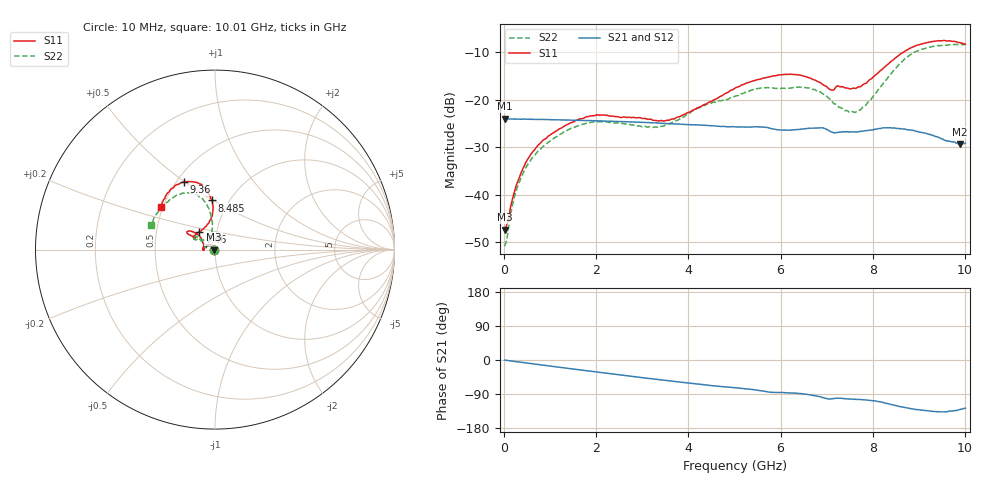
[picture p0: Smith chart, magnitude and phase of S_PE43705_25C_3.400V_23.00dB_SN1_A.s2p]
! Device ID: PE43705
! Serial: 1
! Insertion: A
! Impedance: 50 ohm
! Temp: 25C
! VDD: 3.400V
! Attenuation Step: 23.00dB
#  Hz  S  RI  R  50
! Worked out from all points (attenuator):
!   401 points, 10 MHz to 10.01 GHz, reference 50 ohm
!   highest |S21| = -24.02 dB at 10 MHz (marker M1); lowest = -29.3 dB at 9.885 GHz (marker M2)
!   lowest |S11| = -47.4 dB at 10 MHz (marker M3), VSWR 1.01, Z = 49.6 + j0.0438 ohm
!   |S11| at or under -10 dB: start of sweep to 8.665 GHz
!   |S22| runs from -50.8 to -8.3 dB; largest |S21 - S12| = 0.001
!   S11 on the Smith chart (normalised r, x): 10 MHz: 0.99, +0.00; 7.46 GHz: 0.82, +0.16; 8.485 GHz: 0.83, +0.49; 9.36 GHz: 0.55, +0.50; 10.01 GHz: 0.49, +0.27
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1e7  -0.00426 0.000441  0.0629 -0.000248  0.063 -0.000261  -0.00284 0.000469
2.6e8  -0.00556 0.0111  0.0624 -0.00478  0.0623 -0.00473  -0.00361 0.0104
5.35e8  -0.0124 0.0212  0.0616 -0.00955  0.0616 -0.00946  -0.00964 0.0192
1.01e9  -0.0331 0.0274  0.0592 -0.0173  0.0592 -0.0173  -0.0277 0.0245
1.685e9  -0.0608 0.0173  0.0541 -0.0271  0.0541 -0.0271  -0.0522 0.0168
2.085e9  -0.0685 0.00614  0.0503 -0.0323  0.0503 -0.0322  -0.0581 0.00856
3.36e9  -0.0597 0.00424  0.035 -0.0445  0.0351 -0.0446  -0.05 0.0129
3.86e9  -0.063 0.0271  0.0285 -0.0472  0.0286 -0.0471  -0.0586 0.0278
4.385e9  -0.0727 0.053  0.022 -0.049  0.0221 -0.049  -0.0746 0.0479
5.01e9  -0.0995 0.0874  0.0147 -0.0497  0.0151 -0.0496  -0.0886 0.0634
5.535e9  -0.129 0.1006  0.00857 -0.0511  0.00868 -0.051  -0.1083 0.0743
5.985e9  -0.1513 0.1026  0.0036 -0.0479  0.00359 -0.0478  -0.11 0.0713
6.685e9  -0.1432 0.082  -0.00276 -0.0501  -0.00292 -0.05  -0.1144 0.0587
7.085e9  -0.1096 0.0646  -0.0102 -0.045  -0.0101 -0.0452  -0.0841 0.0555
7.46e9  -0.0883 0.0984  -0.0101 -0.045  -0.0101 -0.0447  -0.0498 0.0575
7.785e9  -0.0449 0.1365  -0.012 -0.0452  -0.0115 -0.0452  -0.0276 0.079
8.36e9  -0.0109 0.244  -0.0223 -0.0455  -0.0223 -0.0456  -0.0198 0.1788
8.485e9  -0.0172 0.2737  -0.0249 -0.0435  -0.025 -0.0436  -0.0289 0.2102
8.885e9  -0.0692 0.3537  -0.03 -0.0367  -0.0295 -0.0365  -0.0908 0.297
9.36e9  -0.1718 0.3752  -0.0296 -0.0283  -0.0297 -0.0284  -0.1986 0.3067
9.885e9  -0.2854 0.2803  -0.0224 -0.0259  -0.0226 -0.0258  -0.3341 0.1874
1.001e10  -0.302 0.2388  -0.0212 -0.0278  -0.0212 -0.0276  -0.358 0.1362
